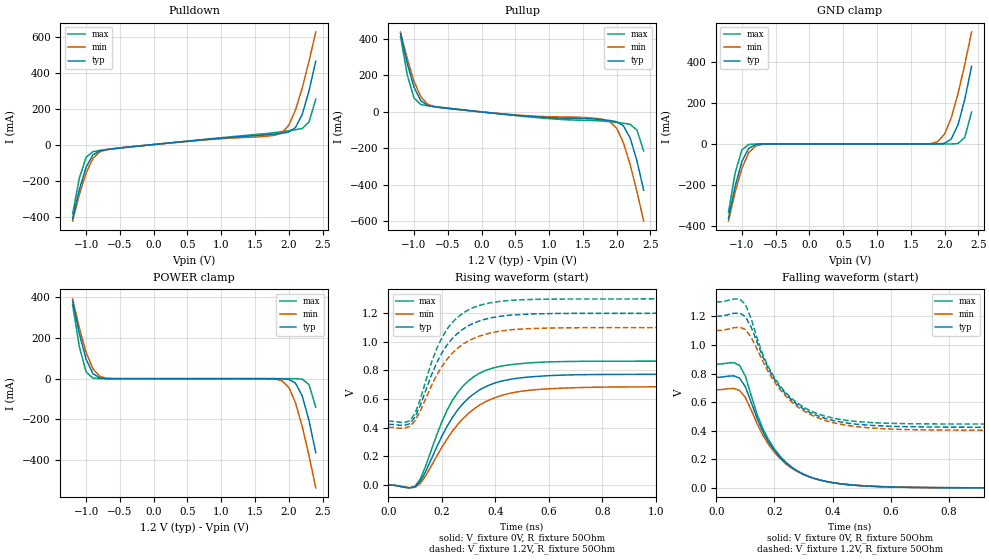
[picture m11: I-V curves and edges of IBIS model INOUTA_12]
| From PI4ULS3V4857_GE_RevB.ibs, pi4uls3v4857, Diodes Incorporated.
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[Model]  INOUTA_12
Model_type  I/O
Vinl = 0.24V
Vinh = 0.96V
Vmeas=0.6
|Variable   typ   min   max
C_comp   4.38p   4.35p   4.41p
[Voltage Range]   1.2   1.1   1.3
[Temperature Range]   40   85   -40
[Pullup Reference]   1.2   1.1   1.3
[Pulldown Reference]   0   0   0
[Power Clamp Reference]   1.2   1.1   1.3
[GND Clamp Reference]   0   0   0
[Driver Schedule]
|Model_Name   Rise_on_dly   Rise_off_dly   Fall_on_dly   Fall_off_dly
IOA_12_1   0.00ns   4.80ns   NA   NA
IOA_12_2   0.00ns   NA   0.00ns   NA
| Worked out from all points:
|   slope of the pulldown table from 0 to 0.18 V, typ, clamps not added: 26.9 ohm
|   slope of the pullup table from 0 to 0.18 V, typ, clamps not added: 26.7 ohm
|   GND clamp passes 1 mA (typ) near -0.72 V on its own axis
|   POWER clamp passes 1 mA (typ) near -0.72 V on its own axis
|   falling waveform, V_fixture 0V, R_fixture 50Ohm: 20-80 % time 135ps typ, 140ps min, 130ps max; typ from 0.773 V to 0.001 V
|   falling waveform, V_fixture 1.2V, R_fixture 50Ohm: 20-80 % time 145ps typ, 156ps min, 136ps max; typ from 1.2 V to 0.424 V
|   rising waveform, V_fixture 0V, R_fixture 50Ohm: 20-80 % time 153ps typ, 172ps min, 132ps max; typ from 0.001 V to 0.773 V
|   rising waveform, V_fixture 1.2V, R_fixture 50Ohm: 20-80 % time 127ps typ, 137ps min, 114ps max; typ from 0.424 V to 1.2 V
[GND Clamp]
-1.2V     -363mA     -377mA     -335mA
-1.1V     -205mA     -235mA     -140mA
-1V       -84.8mA    -118mA     -28.6mA
-900mV    -21.7mA    -42.8mA    -2.29mA
-800mV    -3.31mA    -10.4mA    -51.5uA
1.7V      183nA      121uA      6.42pA
1.9V      214uA      11.7mA     2.28nA
2V        3.47mA     48.5mA     315nA
2.1V      24.8mA     129mA      39.3uA
2.2V      94.6mA     248mA      2.33mA
2.3V      220mA      391mA      33mA
2.4V      380mA      548mA      156mA
[POWER Clamp]
-1.2V     380mA      391mA      362mA
-1.1V     220mA      248mA      156mA
-1V       94.7mA     129mA      33.1mA
-900mV    24.9mA     48.6mA     2.36mA
-800mV    3.5mA      11.7mA     65.4uA
-600mV    27uA       142uA      19.6uA
1.9V      -320uA     -10.4mA    -62.1uA
2V        -3.38mA    -42.8mA    -65.8uA
2.1V      -21.8mA    -118mA     -120uA
2.2V      -84.9mA    -235mA     -2.36mA
2.3V      -205mA     -377mA     -28.7mA
2.4V      -363mA     -535mA     -140mA
[Pulldown]
| Voltage   I(typ)   I(min)  I(max)
-1.2V     -412mA     -425mA     -386mA
-1.1V     -250mA     -278mA     -186mA
-1V       -126mA     -158mA     -70.7mA
-900mV    -58.2mA    -78mA      -39.8mA
-800mV    -35.5mA    -41.4mA    -33.1mA
-400mV    -15.2mA    -14.6mA    -15.6mA
1.9V      62.2mA     65.8mA     71.5mA
2V        69.2mA     107mA      76.8mA
2.1V      94.5mA     192mA      82mA
2.2V      168mA      315mA      89.2mA
2.3V      298mA      463mA      125mA
2.4V      463mA      625mA      252mA
[Pullup]   |Note: Vtable = Vcc - Voutput
| Voltage   I(typ)   I(min)  I(max)
-1.2V     430mA      438mA      413mA
-1.1V     265mA      291mA      203mA
-1V       135mA      168mA      75.7mA
-900mV    61.3mA     83.3mA     40.7mA
-800mV    35.7mA     42.4mA     34mA
0V        3.48nA     37.2nA     15.4pA
1.9V      -47mA      -53.2mA    -53.7mA
2V        -53.9mA    -89.4mA    -57.6mA
2.1V      -76.2mA    -169mA     -61.8mA
2.2V      -143mA     -289mA     -68.2mA
2.3V      -267mA     -436mA     -98.8mA
2.4V      -429mA     -598mA     -214mA
[Falling Waveform]
V_fixture = 0V
V_fixture_min = 0V
V_fixture_max = 0V
R_fixture = 50Ohm
C_fixture = 0F
|   Time   V(typ)   V(min)   V(max)
0s        772.9mV    685.8mV    864.8mV
80ps      768.5mV    682.2mV    857.8mV
100ps     707.5mV    633mV      782.2mV
140ps     487.2mV    451.1mV    516.6mV
160ps     395mV      369.2mV    415.9mV
220ps     212.9mV    204.3mV    220.5mV
280ps     115.7mV    113.5mV    118.2mV
380ps     43.93mV    44.33mV    44.52mV
680ps     3.628mV    3.967mV    3.456mV
1.98ns    698.9uV    664uV      722.5uV
[Falling Waveform]
V_fixture = 1.2V
V_fixture_min = 1.1V
V_fixture_max = 1.3V
R_fixture = 50Ohm
C_fixture = 0F
|   Time   V(typ)   V(min)   V(max)
0s        1.2V       1.1V       1.3V
80ps      1.223V     1.124V     1.322V
100ps     1.198V     1.108V     1.285V
120ps     1.125V     1.054V     1.184V
160ps     917.9mV    885.9mV    932.8mV
220ps     702.1mV    686.7mV    711.8mV
300ps     552.7mV    539.9mV    565mV
400ps     472.7mV    457.5mV    489.8mV
700ps     426.9mV    406.5mV    448.4mV
1.98ns    424.2mV    402.9mV    446.3mV
[Rising Waveform]
V_fixture = 0V
V_fixture_min = 0V
V_fixture_max = 0V
R_fixture = 50Ohm
C_fixture = 0F
|   Time   V(typ)   V(min)   V(max)
0s        698.8uV    663.8uV    722.5uV
100ps     -12.44mV   -16.34mV   -9.06mV
120ps     25.69mV    11.44mV    43.15mV
220ps     411.3mV    322.8mV    523.7mV
260ps     526.1mV    424.3mV    648mV
320ps     637.2mV    531.2mV    756.9mV
400ps     713.2mV    610.6mV    821.1mV
520ps     753mV      659.8mV    851.6mV
720ps     770.1mV    680.5mV    863.4mV
1.98ns    772.9mV    685.8mV    864.8mV
[Rising Waveform]
V_fixture = 1.2V
V_fixture_min = 1.1V
V_fixture_max = 1.3V
R_fixture = 50Ohm
C_fixture = 0F
|   Time   V(typ)   V(min)   V(max)
0s        423.9mV    402.8mV    445.9mV
80ps      428.1mV    408.8mV    447.2mV
100ps     474.6mV    449.1mV    500.6mV
180ps     850mV      763.8mV    949.3mV
220ps     980mV      879.9mV    1.091V
280ps     1.09V      984.6mV    1.202V
360ps     1.157V     1.051V     1.264V
460ps     1.187V     1.084V     1.29V
620ps     1.198V     1.097V     1.298V
1.98ns    1.2V       1.1V       1.3V
[Ramp]
|   typ   min   max
dV/dt_r   0.63/1.02E-10   0.56/1.15E-10   0.70/0.88E-10
dV/dt_f   0.63/1.34E-10   0.56/1.40E-10   0.70/1.30E-10
R_load =   50.0000
